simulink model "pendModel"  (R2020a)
settings: Solver=VariableStepAuto  StartTime=0.0  StopTime=10.0  RelTol=1e-3
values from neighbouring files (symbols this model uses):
  a = 10    [initParams.m]
  b = 1    [initParams.m]
  x0 = [0.2;0.1]    [initParams.m]

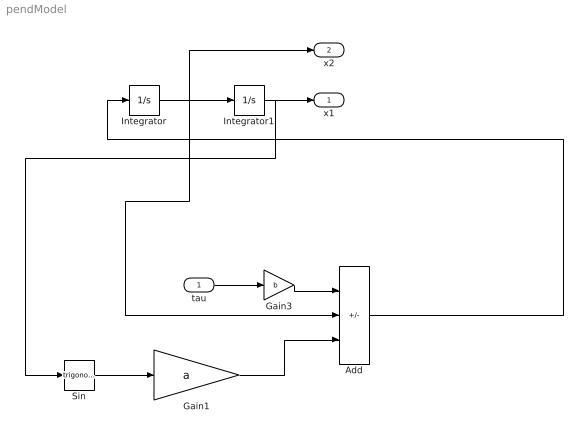
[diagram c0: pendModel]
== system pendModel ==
  tau : Inport
  Add : Sum  Inputs=+--
  Gain1 : Gain  Gain=a
  Gain3 : Gain  Gain=b
  Integrator : Integrator  InitialCondition=x0(2)
  Integrator1 : Integrator  InitialCondition=x0(1)
  Sin : Trigonometry
  x1 : Outport
  x2 : Outport  Port=2
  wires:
  Integrator1/1 -> Sin/1, x1/1
  tau/1 -> Gain3/1
  Integrator/1 -> Add/2, x2/1, Integrator1/1
  Sin/1 -> Gain1/1
  Gain1/1 -> Add/3
  Add/1 -> Integrator/1
  Gain3/1 -> Add/1
